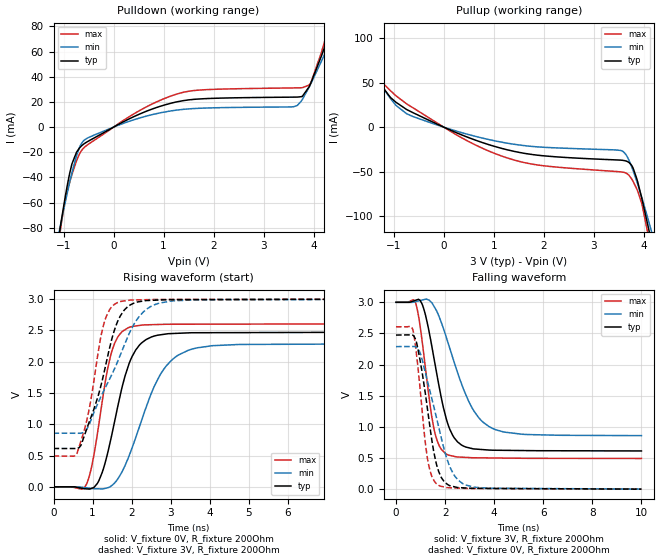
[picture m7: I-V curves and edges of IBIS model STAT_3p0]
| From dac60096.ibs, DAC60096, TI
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|   Model
[Model]   STAT_3p0
Model_type   Output
Polarity   Non-Inverting
Vmeas = 1.5
Vref = 0
Cref = 1pF
Rref = 100000
|   typ   min   max
C_comp   12.144pF   11.345pF   12.754pF
[Voltage Range]   3   2.999   3.001
[Temperature Range]   27   105   -40
[Pullup Reference]   3   2.999   3.001
[Pulldown Reference]   0   0   0
[Power Clamp Reference]   3   2.999   3.001
[GND Clamp Reference]   0   0   0
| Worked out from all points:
|   slope of the pulldown table from 0 to 0.45 V, typ, clamps not added: 49.3 ohm
|   slope of the pullup table from 0 to 0.45 V, typ, clamps not added: 42 ohm
|   falling waveform, V_fixture 3V, R_fixture 200Ohm: 20-80 % time 727ps typ, 1.19ns min, 511ps max; typ from 3 V to 0.614 V
|   rising waveform, V_fixture 0V, R_fixture 200Ohm: 20-80 % time 572ps typ, 858ps min, 420ps max; typ from 0 V to 2.47 V
|   rising waveform, V_fixture 3V, R_fixture 200Ohm: 20-80 % time 623ps typ, 934ps min, 421ps max; typ from 0.613 V to 3 V
|   falling waveform, V_fixture 0V, R_fixture 200Ohm: 20-80 % time 574ps typ, 880ps min, 412ps max; typ from 2.47 V to 0.001 V
[Pulldown]
|   Voltage   I(typ)   I(min)   I(max)
-3V       -639.8mA   -520.6mA   -766.4mA
-1.056V   -77.26mA   -76.95mA   -80.04mA
-975mV    -57.53mA   -61.44mA   -59.82mA
-831mV    -29.12mA   -36.12mA   -37.53mA
-633mV    -14.62mA   -12.51mA   -18.23mA
519mV     10.36mA    7.231mA    13.13mA
1.527V    21.76mA    14.57mA    28.67mA
3.669V    23.87mA    17.15mA    31.19mA
3.777V    24.56mA    22.05mA    31.34mA
3.948V    35.27mA    34.67mA    35.46mA
4.362V    78.89mA    70.4mA     87.48mA
6V        266.5mA    221mA      324.6mA
[Pullup]
|   Voltage   I(typ)   I(min)   I(max)
-3V       245mA      206.1mA    297.4mA
-1.83V    111.2mA    98.6mA     128.5mA
-1.182V   42.04mA    41.54mA    47.49mA
-957mV    28.04mA    24.54mA    35.3mA
-615mV    16.26mA    11.93mA    21.73mA
1.275V    -25.52mA   -18.06mA   -34.7mA
3.579V    -37.29mA   -27.13mA   -50.54mA
3.786V    -45.87mA   -48.71mA   -60.87mA
3.885V    -62.84mA   -65.21mA   -72.7mA
4.092V    -112.7mA   -104.4mA   -122.2mA
4.191V    -138.9mA   -124.5mA   -154.5mA
6V        -667.8mA   -542.1mA   -801.7mA
[Ramp]
R_load = 200
|   typ   min   max
dV/dt_r   1.48421/5.7207e-10   1.37266/8.58185e-10   1.56435/4.19453e-10
dV/dt_f   1.43179/7.26267e-10   1.28381/1.18696e-09   1.5048/5.09918e-10
[Falling Waveform]
V_fixture = 3V
V_fixture_min = 2.999V
V_fixture_max = 3.001V
R_fixture = 200Ohm
C_fixture = 0F
|   Time   V(typ)   V(min)   V(max)
0s        3V         2.999V     3.001V
801.7ps   3.033V     3.012V     2.988V
1.119ns   2.91V      3.042V     2.206V
1.542ns   2.114V     2.94V      980.4mV
1.761ns   1.641V     2.765V     697.7mV
2.018ns   1.177V     2.477V     572.4mV
2.368ns   827mV      2.041V     526.8mV
3.031ns   658.3mV    1.355V     506.4mV
3.926ns   625.9mV    976.6mV    501.1mV
10ns      613.7mV    859.3mV    493mV
[Rising Waveform]
V_fixture = 0V
V_fixture_min = 0V
V_fixture_max = 0V
R_fixture = 200Ohm
C_fixture = 0F
|   Time   V(typ)   V(min)   V(max)
0s        -374.8nV   -47.21nV   -187.5nV
840.6ps   -32.43mV   -14.85mV   37.5mV
985.1ps   -21.37mV   -26.46mV   352.8mV
1.164ns   104.1mV    -31.52mV   1.02V
1.46ns    746.3mV    7.795mV    2.096V
1.908ns   1.921V     455.1mV    2.542V
2.252ns   2.299V     1.059V     2.584V
2.715ns   2.428V     1.776V     2.595V
3.454ns   2.461V     2.184V     2.599V
10ns      2.474V     2.288V     2.607V
[Rising Waveform]
V_fixture = 3V
V_fixture_min = 2.999V
V_fixture_max = 3.001V
R_fixture = 200Ohm
C_fixture = 0F
|   Time   V(typ)   V(min)   V(max)
0s        613.2mV    857.3mV    492.9mV
597.5ps   612.6mV    856.6mV    530.7mV
705.9ps   670.8mV    857.4mV    741.6mV
899.5ps   1.013V     979.1mV    1.203V
1.275ns   1.779V     1.523V     2.576V
1.435ns   2.219V     1.722V     2.831V
1.64ns    2.643V     2.002V     2.946V
2.138ns   2.952V     2.677V     2.987V
2.715ns   2.986V     2.938V     2.994V
10ns      3V         2.999V     3.001V
[Falling Waveform]
|Gnd
V_fixture = 0V
V_fixture_min = 0V
V_fixture_max = 0V
R_fixture = 200Ohm
C_fixture = 0F
|   Time   V(typ)   V(min)   V(max)
0s        2.474V     2.289V     2.607V
696.6ps   2.469V     2.29V      2.545V
900.8ps   2.236V     2.248V     1.934V
1.159ns   1.632V     1.929V     875mV
1.275ns   1.307V     1.743V     509.7mV
1.46ns    787mV      1.453V     205.6mV
1.718ns   309.1mV    1.033V     66.82mV
2.233ns   51.89mV    325mV      22.43mV
2.822ns   19.7mV     69.07mV    12.27mV
10ns      513.9uV    1.473mV    117.9uV
